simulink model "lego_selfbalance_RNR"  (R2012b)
settings: Solver=ode3  SolverMode=SingleTasking  StartTime=0.0  StopTime=100  FixedStep=0.004  MaxStep=TS  RelTol=1e-3
PostLoadFcn:
  | lego2_selfbalance_plant;
  | lego2_selfbalance_controller;
  | lego_selfbalance_simulation;
InitFcn:
  | lego2_selfbalance_plant;
  | lego2_selfbalance_controller;
  | lego_selfbalance_simulation;
  | 
  | lego_drive_selfbalance_InitData.mdl = get_param(bdroot,'Name');
  | lego_drive_selfbalance_InitData.cs = getActiveConfigSet(lego_drive_selfbalance_InitData.mdl);
model workspace: external: MAT-File (data not in the file)
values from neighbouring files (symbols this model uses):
  A1 = [    [lego2_selfbalance_plant.m]
  A2 = [    [lego2_selfbalance_plant.m]
  a_b = 0.8    [lego2_selfbalance_controller.m]
  a_d = 0.8    [lego2_selfbalance_controller.m]
  a_gc = 0.8    [lego2_selfbalance_controller.m]
  a_gd = 0.999    [lego2_selfbalance_controller.m]
  a_r = 0.996    [lego2_selfbalance_controller.m]
  B1 = [    [lego2_selfbalance_plant.m]
  B2 = [    [lego2_selfbalance_plant.m]
  BATTERY = 8000    [lego_selfbalance_simulation.m]
  C1 = eye(4)    [lego2_selfbalance_plant.m]
  C2 = eye(2)    [lego2_selfbalance_plant.m]
  D = 0.04    [lego2_selfbalance_plant.m]
  D1 = zeros(4, 2)    [lego2_selfbalance_plant.m]
  D2 = zeros(2)    [lego2_selfbalance_plant.m]
  GYRO0 = 600    [lego_selfbalance_simulation.m]
  k_f = KK(1, 1:4)    [lego2_selfbalance_controller.m]
  k_i = KK(1, 5)    [lego2_selfbalance_controller.m]
  k_sync = 0.35    [lego2_selfbalance_controller.m]
  pwm_gain = 1    [lego2_selfbalance_controller.m]
  pwm_offset = 0    [lego2_selfbalance_controller.m]
  R = 0.03    [lego2_selfbalance_plant.m]
  START_POS = [100, 100]    [lego_selfbalance_simulation.m]
  time_start = 4000    [lego2_selfbalance_controller.m]
  TS = 0.001    [lego_selfbalance_simulation.m]
  ts1 = 0.004    [lego2_selfbalance_controller.m]
  W = 0.068    [lego2_selfbalance_plant.m]
  X1IV = [    [lego_selfbalance_simulation.m]
  X2IV = [    [lego_selfbalance_simulation.m]
undefined symbols (not defined in the file or in its folder): A, DiscIntNeverNeededParam, Raw
libraries: legonxtlib x8, simulink x4

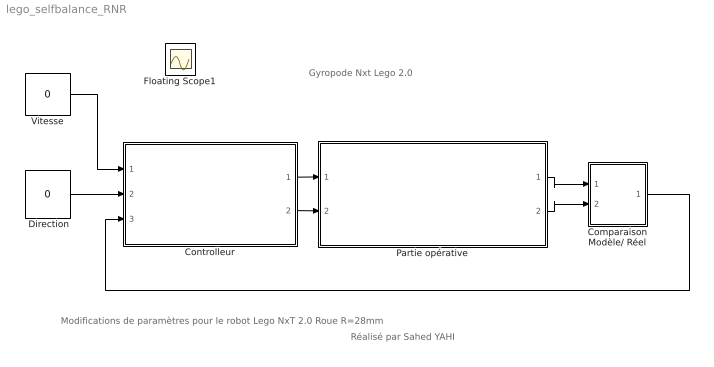
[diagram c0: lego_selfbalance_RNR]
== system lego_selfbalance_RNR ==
  note: Modifications de paramètres pour le robot Lego NxT 2.0 Roue R=28mm
  note: Réalisé par Sahed YAHI
  note: Gyropode Nxt Lego 2.0
  "   Vitesse   " : Constant  Value=0  OutDataTypeStr=single  SampleTime=4*TS
  " Direction" : Constant  Value=0  OutDataTypeStr=single  SampleTime=4*TS
  Comparaison Modèle/ Réel : Subsystem
  Controlleur : Subsystem  TreatAsAtomicUnit=on
  Partie opérative : Subsystem
  Floating Scope1 : Scope
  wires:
  "   Vitesse   "/1 -> Controlleur/1(Speed)
  " Direction"/1 -> Controlleur/2(Turn Angle)
  Controlleur/1(Right Wheel Speed) -> Partie opérative/1(R. Wheel Speed)
  Controlleur/2(Left Wheel Speed) -> Partie opérative/2(L. Wheel Speed)
  Partie opérative/1(Simulated Sensor Signals) -> Comparaison Modèle/ Réel/1(In1)
  Partie opérative/2(Actual Sensor Signals) -> Comparaison Modèle/ Réel/2(In2)
  Comparaison Modèle/ Réel/1(Out1) -> Controlleur/3(Sensor Signals)

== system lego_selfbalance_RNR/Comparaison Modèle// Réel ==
  In1 : Inport
  In2 : Inport  Port=2
  Comparaison Modèle/ Réel : simulink/Signal Routing/Environment Controller
  Out1 : Outport
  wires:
  Comparaison Modèle/ Réel/1 -> Out1/1
  In1/1 -> Comparaison Modèle/ Réel/1
  In2/1 -> Comparaison Modèle/ Réel/2

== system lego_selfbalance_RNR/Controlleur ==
  Speed : Inport
  Turn Angle : Inport  Port=2
  Sensor Signals : Inport  Port=3
  Balance and Drive Control : Subsystem
  Compare To Constant : simulink/Logic and Bit Operations/Compare To Constant  relop=>=  const=time_start  OutDataTypeStr=boolean
  Demux : Demux  Outputs=5
  Gyro Calibration : Subsystem  TreatAsAtomicUnit=on
  Logical Operator : Logic  Operator=NOT  AllPortsSameDT=off  OutDataTypeStr=boolean
  Right Wheel Speed : Outport
  Left Wheel Speed : Outport  Port=2
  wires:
  Compare To Constant/1 -> Logical Operator/1, Balance and Drive Control/Enable
  Gyro Calibration/1(Gyro Offset) -> Balance and Drive Control/1(Gyro Offset)
  Logical Operator/1 -> Gyro Calibration/Enable
  Sensor Signals/1 -> Demux/1
  Demux/4 -> Gyro Calibration/1(Gyro), Balance and Drive Control/2(Gyro)
  Speed/1 -> Balance and Drive Control/3(Speed)
  Turn Angle/1 -> Balance and Drive Control/4(Turn Angle)
  Demux/5 -> Balance and Drive Control/7(Battery)
  Demux/3 -> Balance and Drive Control/6(L. Wheel Rotation)
  Demux/2 -> Balance and Drive Control/5(R. Wheel Rotation)
  Demux/1 -> Compare To Constant/1
  Balance and Drive Control/1(R. Wheel Speed) -> Right Wheel Speed/1
  Balance and Drive Control/2(L. Wheel Speed) -> Left Wheel Speed/1

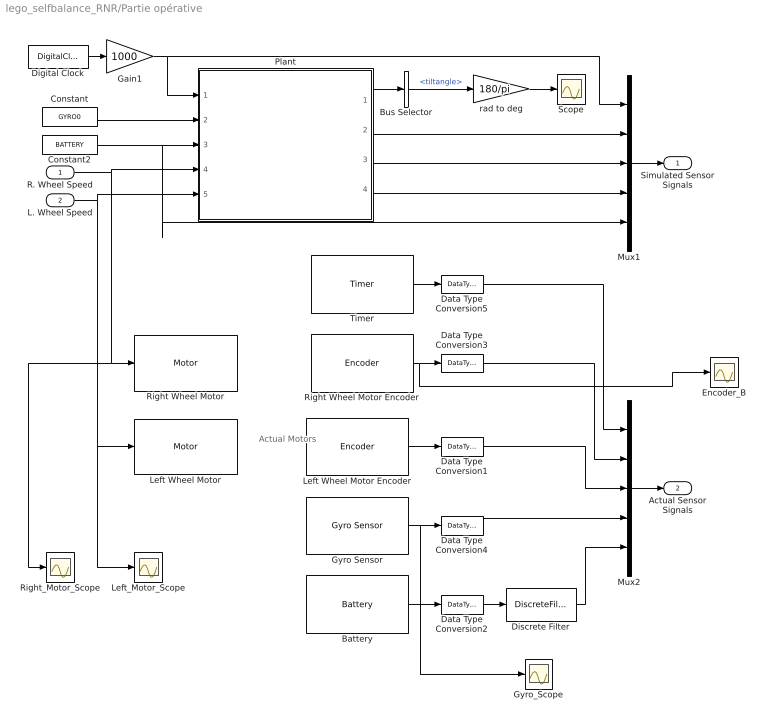
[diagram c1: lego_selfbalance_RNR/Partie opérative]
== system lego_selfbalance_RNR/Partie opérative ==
  note: Actual Motors
  R. Wheel Speed : Inport
  L. Wheel Speed : Inport  Port=2
  Battery : legonxtlib/Battery  sampleTime=ts1
  Bus Selector : BusSelector  OutputSignals=tiltangle
  Constant : Constant  Value=GYRO0  OutDataTypeStr=single
  Constant2 : Constant  Value=BATTERY  OutDataTypeStr=single
  Data Type Conversion{1..5} (5 alike) : DataTypeConversion  OutDataTypeStr=single  RndMeth=Simplest
  Digital Clock : DigitalClock  SampleTime=4*TS
  Discrete Filter : DiscreteFilter  Numerator=[1-a_b]  Denominator=[1 -a_b]
  Encoder_B : Scope
  Gain1 : Gain  Gain=1000  OutDataTypeStr=single
  Gyro Sensor : legonxtlib/Gyro Sensor  portNumber=4  outputMode=Raw A/D (0 - 1023)  offset=600  sampleTime=ts1
  Gyro_Scope : Scope
  Left Wheel Motor : legonxtlib/Motor  sportNumber=C  sstopAction=Brake
  Left Wheel Motor Encoder : legonxtlib/Encoder  portNumber=C  opMode=No reset  sampleTime=ts1
  Left_Motor_Scope : Scope
  Mux1 : Mux  Inputs=5
  Mux2 : Mux  Inputs=5
  Plant : Subsystem
  Right Wheel Motor : legonxtlib/Motor  sportNumber=B  sstopAction=Brake
  Right Wheel Motor Encoder : legonxtlib/Encoder  portNumber=B  opMode=No reset  sampleTime=ts1
  Right_Motor_Scope : Scope
  Scope : Scope
  Timer : legonxtlib/Timer  sampleTime=ts1
  rad to deg : Gain  Gain=180/pi
  Simulated Sensor Signals : Outport
  Actual Sensor Signals : Outport  Port=2
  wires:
  Data Type Conversion5/1 -> Mux2/1
  Timer/1 -> Data Type Conversion5/1
  Data Type Conversion4/1 -> Mux2/4
  Data Type Conversion1/1 -> Mux2/3
  Data Type Conversion3/1 -> Mux2/2
  Mux2/1 -> Actual Sensor Signals/1
  Left Wheel Motor Encoder/1 -> Data Type Conversion1/1
  Right Wheel Motor Encoder/1 -> Encoder_B/1, Data Type Conversion3/1
  Battery/1 -> Data Type Conversion2/1
  Data Type Conversion2/1 -> Discrete Filter/1
  Discrete Filter/1 -> Mux2/5
  Gyro Sensor/1 -> Gyro_Scope/1, Data Type Conversion4/1
  L. Wheel Speed/1 -> Plant/5(L. Wheel Speed), Left_Motor_Scope/1, Left Wheel Motor/1
  Mux1/1 -> Simulated Sensor Signals/1
  Plant/3(L. Wheel Rotation) -> Mux1/3
  Constant2/1 -> Mux1/5, Plant/3(Battery)
  Plant/2(R. Wheel Rotation) -> Mux1/2
  Plant/4(Gyro) -> Mux1/4
  Digital Clock/1 -> Gain1/1
  Gain1/1 -> Mux1/1, Plant/1(Clock)
  rad to deg/1 -> Scope/1
  Plant/1(Vertical Displacement) -> Bus Selector/1
  Bus Selector/1 -> rad to deg/1  "<tiltangle>"
  Constant/1 -> Plant/2(Gyro Offset)
  R. Wheel Speed/1 -> Plant/4(R. Wheel Speed), Right Wheel Motor/1, Right_Motor_Scope/1

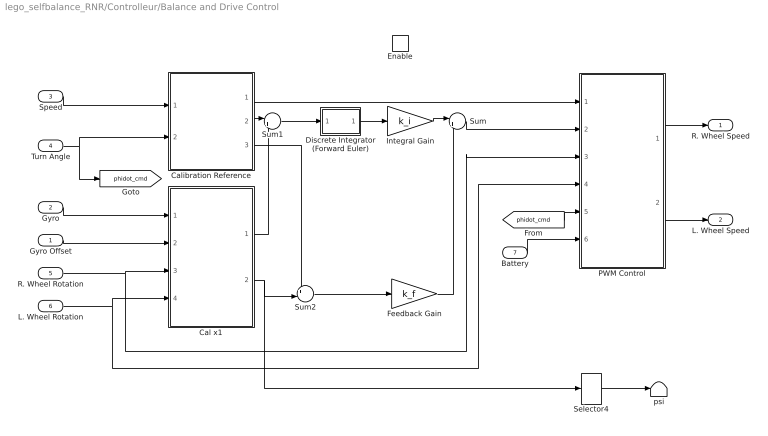
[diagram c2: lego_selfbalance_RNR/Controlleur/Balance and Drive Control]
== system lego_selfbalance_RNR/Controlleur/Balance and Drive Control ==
  Gyro Offset : Inport
  Gyro : Inport  Port=2
  Speed : Inport  Port=3
  Turn Angle : Inport  Port=4
  R. Wheel Rotation : Inport  Port=5
  L. Wheel Rotation : Inport  Port=6
  Battery : Inport  Port=7
  Enable : EnablePort
  Cal x1 : Subsystem
  Calibration Reference : Subsystem
  Discrete Integrator (Forward Euler) : Subsystem
  Feedback Gain : Gain  Gain=k_f  Multiplication=Matrix(K*u)
  Integral Gain : Gain  Gain=k_i  Multiplication=Matrix(K*u)
  PWM Control : Subsystem
  Selector4 : Selector  InputPortWidth=4  IndexOptions=Index vector (dialog)  Indices=2  OutputSizes=1
  Sum : Sum  Inputs=|++
  Sum1 : Sum  Inputs=|+-
  Sum2 : Sum  Inputs=+-|
  psi : Terminator
  R. Wheel Speed : Outport
  L. Wheel Speed : Outport  Port=2
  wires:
  [phidot_cmd] -> PWM Control/5(phidot_cmd)
  Selector4/1 -> psi/1
  Calibration Reference/3(x1_ref) -> Sum2/1
  Sum2/1 -> Feedback Gain/1
  Cal x1/2(x1) -> Selector4/1, Sum2/2
  Integral Gain/1 -> Sum/1
  Discrete Integrator (Forward Euler)/1(Out) -> Integral Gain/1
  Sum1/1 -> Discrete Integrator (Forward Euler)/1(In)
  Cal x1/1(theta) -> Sum1/2
  Calibration Reference/2(theta_ref) -> Sum1/1
  Feedback Gain/1 -> Sum/2
  L. Wheel Rotation/1 -> PWM Control/4(theta_l), Cal x1/4(L. Wheel Rotation)
  Battery/1 -> PWM Control/6(Battery)
  Sum/1 -> PWM Control/2(Voltage)
  Turn Angle/1 -> [phidot_cmd], Calibration Reference/2(Turn Angle)
  Speed/1 -> Calibration Reference/1(Speed)
  Calibration Reference/1(pwm_turn) -> PWM Control/1(pwm_turn)
  PWM Control/1(pwm_r) -> R. Wheel Speed/1
  PWM Control/2(pwm_l) -> L. Wheel Speed/1
  R. Wheel Rotation/1 -> PWM Control/3(theta_r), Cal x1/3(R. Wheel Rotation)
  Gyro/1 -> Cal x1/1(Gyro)
  Gyro Offset/1 -> Cal x1/2(Gyro Offset)

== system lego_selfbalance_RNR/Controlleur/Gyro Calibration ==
  note: Calculate gyro offset
  Gyro : Inport
  Enable : EnablePort
  Constant : Constant  Value=440  OutDataTypeStr=uint32  SampleTime=0.2
  Gain2 : Gain  Gain=1-a_gc
  Gain3 : Gain  Gain=a_gc
  Speaker : legonxtlib/Speaker  sinputMode=Frequency only  sspeakerFreq=100  sspeakerVolume=80  sspeakerDuration=100
  Sum1 : Sum  Inputs=|++
  Unit Delay : UnitDelay  SampleTime=-1
  Gyro Offset : Outport
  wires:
  Gain3/1 -> Sum1/2
  Unit Delay/1 -> Gain3/1
  Sum1/1 -> Unit Delay/1, Gyro Offset/1
  Gain2/1 -> Sum1/1
  Gyro/1 -> Gain2/1
  Constant/1 -> Speaker/1

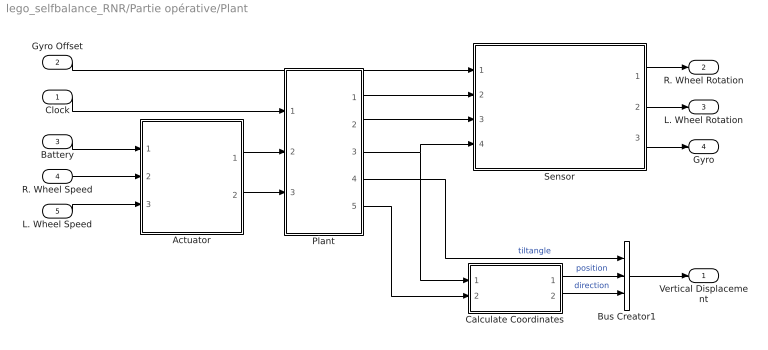
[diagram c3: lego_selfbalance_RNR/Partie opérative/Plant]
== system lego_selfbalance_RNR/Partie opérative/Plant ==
  Clock : Inport
  Gyro Offset : Inport  Port=2
  Battery : Inport  Port=3
  R. Wheel Speed : Inport  Port=4
  L. Wheel Speed : Inport  Port=5
  Actuator : Subsystem
  Bus Creator1 : BusCreator  Inputs=3
  Calculate Coordinates : Subsystem
  Plant : Subsystem
  Sensor : Subsystem
  Vertical Displacement : Outport
  R. Wheel Rotation : Outport  Port=2
  L. Wheel Rotation : Outport  Port=3
  Gyro : Outport  Port=4
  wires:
  Clock/1 -> Plant/1(Clock)
  Plant/4(psi) -> Bus Creator1/1  "tiltangle"
  Bus Creator1/1 -> Vertical Displacement/1
  Calculate Coordinates/2(direction) -> Bus Creator1/3  "direction"
  Calculate Coordinates/1(position) -> Bus Creator1/2  "position"
  Plant/3(phi) -> Calculate Coordinates/1(phi), Sensor/4(phi)
  L. Wheel Speed/1 -> Actuator/3(L. Wheel Speed)
  Plant/5(thetadot) -> Calculate Coordinates/2(thetadot)
  Sensor/3(Gyro) -> Gyro/1
  R. Wheel Speed/1 -> Actuator/2(R. Wheel Speed)
  Sensor/2(L. Wheel Rotation) -> L. Wheel Rotation/1
  Sensor/1(R. Wheel Rotation) -> R. Wheel Rotation/1
  Gyro Offset/1 -> Sensor/1(Gyro Offset)
  Battery/1 -> Actuator/1(Battery)
  Plant/1(theta) -> Sensor/2(theta)
  Plant/2(psidot) -> Sensor/3(psidot)
  Actuator/2(vol_l) -> Plant/3(vol_l)
  Actuator/1(vol_r) -> Plant/2(vol_r)

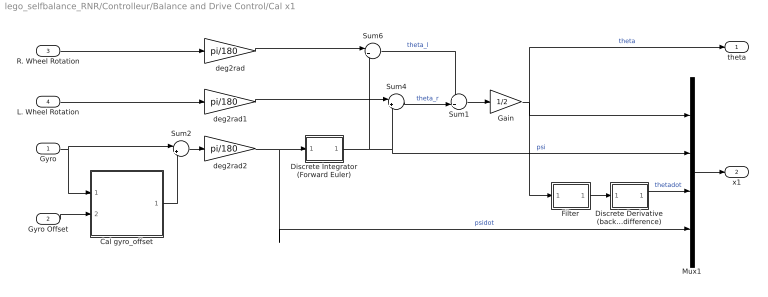
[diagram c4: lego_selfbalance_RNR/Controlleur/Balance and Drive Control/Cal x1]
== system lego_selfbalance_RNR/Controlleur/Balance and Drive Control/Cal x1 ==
  Gyro : Inport
  Gyro Offset : Inport  Port=2
  R. Wheel Rotation : Inport  Port=3
  L. Wheel Rotation : Inport  Port=4
  Cal gyro_offset : Subsystem
  Discrete Derivative (backward difference) : Subsystem
  Discrete Integrator (Forward Euler) : Subsystem
  Filter : Subsystem
  Gain : Gain  Gain=1/2
  Mux1 : Mux
  Sum1 : Sum  Inputs=++|
  Sum2 : Sum  Inputs=|+-
  Sum4 : Sum  Inputs=|++
  Sum6 : Sum  Inputs=|++
  deg2rad : Gain  Gain=pi/180
  deg2rad1 : Gain  Gain=pi/180
  deg2rad2 : Gain  Gain=pi/180
  theta : Outport
  x1 : Outport  Port=2
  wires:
  Gain/1 -> Mux1/1, theta/1, Filter/1(In)  "theta"
  Filter/1(Out) -> Discrete Derivative (backward difference)/1(In)
  deg2rad2/1 -> Mux1/4, Discrete Integrator (Forward Euler)/1(in)  "psidot"
  Sum1/1 -> Gain/1
  Sum4/1 -> Sum1/2  "theta_r"
  Sum6/1 -> Sum1/1  "theta_l"
  Discrete Derivative (backward difference)/1(Out) -> Mux1/3  "thetadot"
  L. Wheel Rotation/1 -> deg2rad1/1
  R. Wheel Rotation/1 -> deg2rad/1
  deg2rad/1 -> Sum6/1
  Discrete Integrator (Forward Euler)/1(out) -> Mux1/2, Sum4/2, Sum6/2  "psi"
  Mux1/1 -> x1/1
  deg2rad1/1 -> Sum4/1
  Gyro/1 -> Sum2/1, Cal gyro_offset/1(Gyro)
  Sum2/1 -> deg2rad2/1
  Cal gyro_offset/1(Gyro Offset) -> Sum2/2
  Gyro Offset/1 -> Cal gyro_offset/2(Gyro Offset 0)

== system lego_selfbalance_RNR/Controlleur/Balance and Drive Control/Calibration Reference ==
  note: thetadot_cmd should be between 0 and 7.5
  note: phidot_cmd should be between 0 and 25
  Speed : Inport
  Turn Angle : Inport  Port=2
  Constant2 : Constant  Value=0  VectorParams1D=off  OutDataTypeStr=single
  Constant3 : Constant  Value=0  VectorParams1D=off  OutDataTypeStr=single
  Discrete Integrator (Forward Euler) : Subsystem
  Filter : Subsystem
  Mux : Mux
  pwm_turn : Outport
  theta_ref : Outport  Port=2
  x1_ref : Outport  Port=3
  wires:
  Filter/1(out) -> Mux/3, Discrete Integrator (Forward Euler)/1(in)  "thetadot_ref"
  Constant3/1 -> Mux/4  "psidot_ref"
  Constant2/1 -> Mux/2  "psi_ref"
  Discrete Integrator (Forward Euler)/1(out) -> Mux/1, theta_ref/1  "theta_ref"
  Mux/1 -> x1_ref/1
  Turn Angle/1 -> pwm_turn/1
  Speed/1 -> Filter/1(in)

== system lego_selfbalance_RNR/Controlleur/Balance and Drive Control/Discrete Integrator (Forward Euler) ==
  In : Inport
  Gain : Gain  Gain=ts1
  Sum : Sum  Inputs=|++
  Unit Delay : UnitDelay  SampleTime=-1
  Out : Outport
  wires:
  In/1 -> Gain/1
  Sum/1 -> Unit Delay/1
  Gain/1 -> Sum/1
  Unit Delay/1 -> Out/1, Sum/2

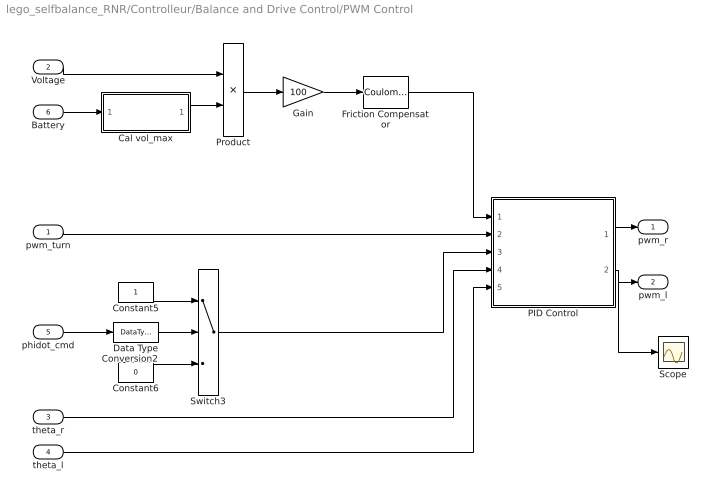
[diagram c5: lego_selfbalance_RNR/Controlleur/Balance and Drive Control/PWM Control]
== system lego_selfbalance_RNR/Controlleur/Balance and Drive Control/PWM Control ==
  pwm_turn : Inport
  Voltage : Inport  Port=2
  theta_r : Inport  Port=3
  theta_l : Inport  Port=4
  phidot_cmd : Inport  Port=5
  Battery : Inport  Port=6
  Cal vol_max : Subsystem
  Constant5 : Constant  OutDataTypeStr=boolean
  Constant6 : Constant  Value=0  OutDataTypeStr=boolean
  Data Type Conversion2 : DataTypeConversion  OutDataTypeStr=int8  RndMeth=Simplest
  Friction Compensator : simulink/Discontinuities/Coulomb & Viscous Friction  offset=pwm_offset  gain=pwm_gain
  Gain : Gain  Gain=100
  PID Control : Subsystem
  Product : Product  Inputs=*/  RndMeth=Simplest
  Scope : Scope
  Switch3 : Switch  Criteria=u2 ~= 0
  pwm_r : Outport
  pwm_l : Outport  Port=2
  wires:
  Data Type Conversion2/1 -> Switch3/2
  phidot_cmd/1 -> Data Type Conversion2/1
  Constant6/1 -> Switch3/3
  Constant5/1 -> Switch3/1
  theta_l/1 -> PID Control/5(In5)
  theta_r/1 -> PID Control/4(In4)
  Cal vol_max/1(vol_max) -> Product/2
  Battery/1 -> Cal vol_max/1(battery)
  Product/1 -> Gain/1
  Voltage/1 -> Product/1
  Gain/1 -> Friction Compensator/1
  PID Control/1(pwm_r) -> pwm_r/1
  Friction Compensator/1 -> PID Control/1(In1)
  PID Control/2(pwm_l) -> Scope/1, pwm_l/1
  pwm_turn/1 -> PID Control/2(In2)
  Switch3/1 -> PID Control/3(In3)

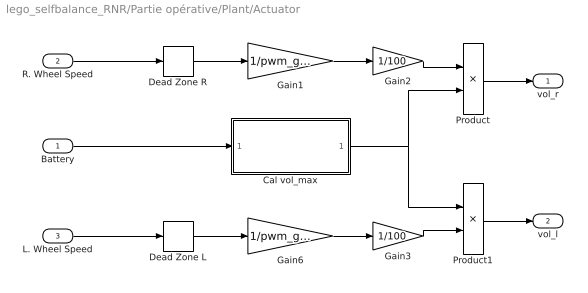
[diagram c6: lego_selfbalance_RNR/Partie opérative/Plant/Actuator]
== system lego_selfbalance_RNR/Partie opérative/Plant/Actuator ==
  Battery : Inport
  R. Wheel Speed : Inport  Port=2
  L. Wheel Speed : Inport  Port=3
  Cal vol_max : Subsystem
  Dead Zone L : DeadZone  LowerValue=-pwm_offset  UpperValue=pwm_offset
  Dead Zone R : DeadZone  LowerValue=-pwm_offset  UpperValue=pwm_offset
  Gain1 : Gain  Gain=1/pwm_gain
  Gain2 : Gain  Gain=1/100
  Gain3 : Gain  Gain=1/100
  Gain6 : Gain  Gain=1/pwm_gain
  Product : Product  RndMeth=Simplest
  Product1 : Product  RndMeth=Simplest
  vol_r : Outport
  vol_l : Outport  Port=2
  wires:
  Battery/1 -> Cal vol_max/1(Battery)
  Cal vol_max/1(vol_max) -> Product1/1, Product/2
  Dead Zone R/1 -> Gain1/1
  Product1/1 -> vol_l/1
  Gain3/1 -> Product1/2
  Product/1 -> vol_r/1
  Gain2/1 -> Product/1
  Gain6/1 -> Gain3/1
  Gain1/1 -> Gain2/1
  L. Wheel Speed/1 -> Dead Zone L/1
  R. Wheel Speed/1 -> Dead Zone R/1
  Dead Zone L/1 -> Gain6/1

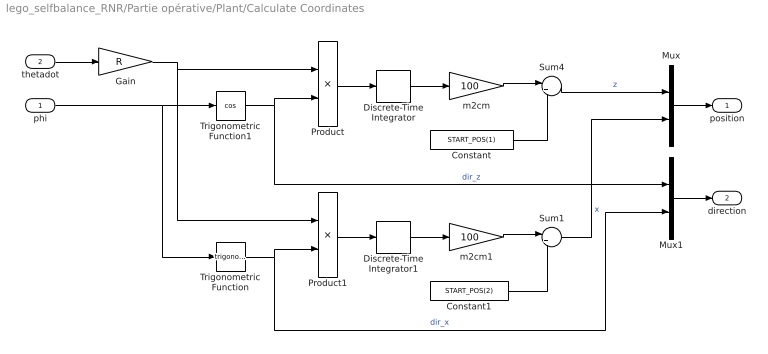
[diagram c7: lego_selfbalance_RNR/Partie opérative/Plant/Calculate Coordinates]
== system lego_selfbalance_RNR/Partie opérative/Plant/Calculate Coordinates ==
  phi : Inport
  thetadot : Inport  Port=2
  Constant : Constant  Value=START_POS(1)  OutDataTypeStr=double
  Constant1 : Constant  Value=START_POS(2)  OutDataTypeStr=double
  Discrete-Time Integrator : DiscreteIntegrator  SampleTime=4*TS  ICPrevOutput=DiscIntNeverNeededParam  ICPrevScaledInput=DiscIntNeverNeededParam
  Discrete-Time Integrator1 : DiscreteIntegrator  SampleTime=4*TS  ICPrevOutput=DiscIntNeverNeededParam  ICPrevScaledInput=DiscIntNeverNeededParam
  Gain : Gain  Gain=R
  Mux : Mux  Inputs=2
  Mux1 : Mux  Inputs=2
  Product : Product  OutDataTypeStr=double  RndMeth=Simplest
  Product1 : Product  OutDataTypeStr=double  RndMeth=Simplest
  Sum1 : Sum  Inputs=|++
  Sum4 : Sum  Inputs=|++
  Trigonometric Function : Trigonometry
  Trigonometric Function1 : Trigonometry  Operator=cos
  m2cm : Gain  Gain=100
  m2cm1 : Gain  Gain=100
  position : Outport
  direction : Outport  Port=2
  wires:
  Mux1/1 -> direction/1
  Mux/1 -> position/1
  Sum1/1 -> Mux/2  "x"
  Constant1/1 -> Sum1/2
  m2cm1/1 -> Sum1/1
  Constant/1 -> Sum4/2
  Sum4/1 -> Mux/1  "z"
  m2cm/1 -> Sum4/1
  Gain/1 -> Product/1, Product1/1
  Discrete-Time Integrator1/1 -> m2cm1/1
  Discrete-Time Integrator/1 -> m2cm/1
  phi/1 -> Trigonometric Function/1, Trigonometric Function1/1
  thetadot/1 -> Gain/1
  Trigonometric Function1/1 -> Mux1/1, Product/2  "dir_z"
  Product/1 -> Discrete-Time Integrator/1
  Trigonometric Function/1 -> Mux1/2, Product1/2  "dir_x"
  Product1/1 -> Discrete-Time Integrator1/1

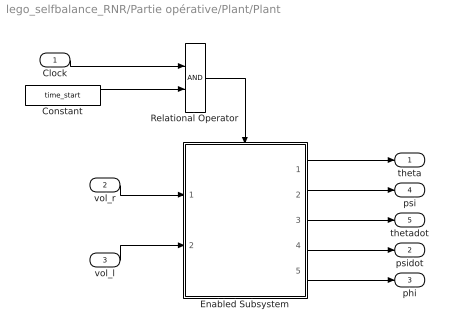
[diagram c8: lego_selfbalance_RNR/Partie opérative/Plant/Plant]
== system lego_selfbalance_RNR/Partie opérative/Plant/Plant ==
  Clock : Inport
  vol_r : Inport  Port=2
  vol_l : Inport  Port=3
  Constant : Constant  Value=time_start  OutDataTypeStr=single
  Enabled Subsystem : Subsystem  TreatAsAtomicUnit=on
  Relational Operator : RelationalOperator  OutDataTypeStr=boolean
  theta : Outport
  psidot : Outport  Port=2
  phi : Outport  Port=3
  psi : Outport  Port=4
  thetadot : Outport  Port=5
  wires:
  Enabled Subsystem/4(psidot) -> psidot/1
  Enabled Subsystem/5(phi) -> phi/1
  Enabled Subsystem/2(psi) -> psi/1
  Enabled Subsystem/3(thetadot) -> thetadot/1
  Enabled Subsystem/1(theta) -> theta/1
  Constant/1 -> Relational Operator/2
  Clock/1 -> Relational Operator/1
  Relational Operator/1 -> Enabled Subsystem/Enable
  vol_l/1 -> Enabled Subsystem/2(vol_l)
  vol_r/1 -> Enabled Subsystem/1(vol_r)

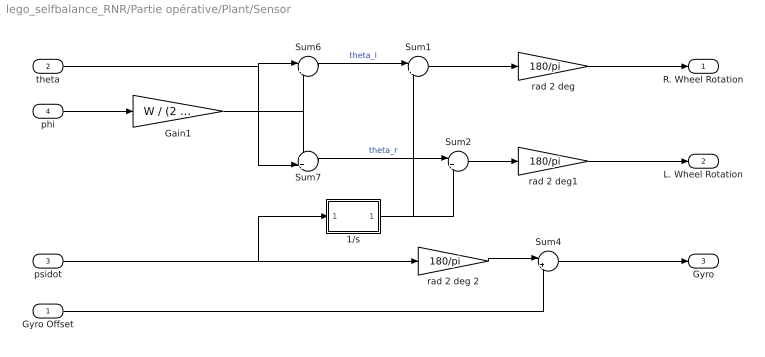
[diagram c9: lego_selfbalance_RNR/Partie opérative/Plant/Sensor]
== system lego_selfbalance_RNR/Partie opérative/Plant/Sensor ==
  Gyro Offset : Inport
  theta : Inport  Port=2
  psidot : Inport  Port=3
  phi : Inport  Port=4
  1/s : Subsystem
  Gain1 : Gain  Gain=W / (2 * R)
  Sum1 : Sum  Inputs=|+-
  Sum2 : Sum  Inputs=|+-
  Sum4 : Sum  Inputs=|++
  Sum6 : Sum  Inputs=|+-
  Sum7 : Sum  Inputs=++|
  rad 2 deg : Gain  Gain=180/pi  OutDataTypeStr=single
  rad 2 deg 2 : Gain  Gain=180/pi
  rad 2 deg1 : Gain  Gain=180/pi  OutDataTypeStr=single
  R. Wheel Rotation : Outport
  L. Wheel Rotation : Outport  Port=2
  Gyro : Outport  Port=3
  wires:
  1/s/1(Out1) -> Sum1/2, Sum2/2
  Sum6/1 -> Sum1/1  "theta_l"
  rad 2 deg1/1 -> L. Wheel Rotation/1
  rad 2 deg/1 -> R. Wheel Rotation/1
  Sum2/1 -> rad 2 deg1/1
  psidot/1 -> 1/s/1(In1), rad 2 deg 2/1
  Sum1/1 -> rad 2 deg/1
  Gain1/1 -> Sum6/2, Sum7/1
  phi/1 -> Gain1/1
  theta/1 -> Sum6/1, Sum7/2
  rad 2 deg 2/1 -> Sum4/1
  Sum7/1 -> Sum2/1  "theta_r"
  Gyro Offset/1 -> Sum4/2
  Sum4/1 -> Gyro/1

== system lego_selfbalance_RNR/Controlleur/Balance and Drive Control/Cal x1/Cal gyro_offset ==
  Gyro : Inport
  Gyro Offset 0 : Inport  Port=2
  Gain1 : Gain  Gain=1-a_gd
  Gain4 : Gain  Gain=a_gd
  Sum2 : Sum  Inputs=|++
  Unit Delay External IC : simulink/Additional Math & Discrete/Additional Discrete/Unit Delay External IC  tsamp=-1
  Gyro Offset : Outport
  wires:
  Gyro/1 -> Gain1/1
  Gyro Offset 0/1 -> Unit Delay External IC/2
  Gain1/1 -> Sum2/1
  Sum2/1 -> Gyro Offset/1, Unit Delay External IC/1
  Unit Delay External IC/1 -> Gain4/1
  Gain4/1 -> Sum2/2

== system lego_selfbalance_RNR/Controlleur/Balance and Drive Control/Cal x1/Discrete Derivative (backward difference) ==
  In : Inport
  Gain : Gain  Gain=1/ts1
  Sum : Sum  Inputs=|+-
  Unit Delay : UnitDelay  SampleTime=-1
  Out : Outport
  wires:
  Gain/1 -> Out/1
  In/1 -> Sum/1, Unit Delay/1
  Unit Delay/1 -> Sum/2
  Sum/1 -> Gain/1

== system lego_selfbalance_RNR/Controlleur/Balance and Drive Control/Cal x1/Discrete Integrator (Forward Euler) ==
  in : Inport
  Gain : Gain  Gain=ts1
  Sum : Sum  Inputs=|++
  Unit Delay : UnitDelay  SampleTime=-1
  out : Outport
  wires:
  Unit Delay/1 -> Sum/2, out/1
  Gain/1 -> Sum/1
  Sum/1 -> Unit Delay/1
  in/1 -> Gain/1

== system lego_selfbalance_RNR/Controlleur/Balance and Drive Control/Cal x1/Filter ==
  In : Inport
  Gain2 : Gain  Gain=a_d
  Gain3 : Gain  Gain=1-a_d
  Sum : Sum  Inputs=|++
  Unit Delay : UnitDelay  SampleTime=-1
  Out : Outport
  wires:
  In/1 -> Gain3/1
  Gain3/1 -> Sum/1
  Gain2/1 -> Sum/2
  Unit Delay/1 -> Gain2/1
  Sum/1 -> Out/1, Unit Delay/1

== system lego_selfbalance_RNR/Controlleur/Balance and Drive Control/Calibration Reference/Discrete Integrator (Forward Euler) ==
  in : Inport
  Gain : Gain  Gain=ts1
  Sum : Sum  Inputs=|++
  Unit Delay : UnitDelay  SampleTime=-1
  out : Outport
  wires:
  in/1 -> Gain/1
  Sum/1 -> Unit Delay/1
  Gain/1 -> Sum/1
  Unit Delay/1 -> out/1, Sum/2

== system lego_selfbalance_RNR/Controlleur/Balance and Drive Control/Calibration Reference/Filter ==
  note: Filter Function: 1-a_r ---------------- 1-a_r*z^(-1)
  in : Inport
  Gain2 : Gain  Gain=a_r
  Gain3 : Gain  Gain=1-a_r
  Sum : Sum  Inputs=|++
  Unit Delay : UnitDelay  SampleTime=-1
  out : Outport
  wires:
  in/1 -> Gain3/1
  Gain3/1 -> Sum/1
  Gain2/1 -> Sum/2
  Unit Delay/1 -> Gain2/1
  Sum/1 -> out/1, Unit Delay/1

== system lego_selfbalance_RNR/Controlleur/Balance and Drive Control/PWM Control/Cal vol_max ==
  battery : Inport
  Constant : Constant  Value=0.625  OutDataTypeStr=single
  Gain3 : Gain  Gain=0.001089
  Sum2 : Sum  Inputs=|+-
  vol_max : Outport
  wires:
  Gain3/1 -> Sum2/1
  Sum2/1 -> vol_max/1
  Constant/1 -> Sum2/2
  battery/1 -> Gain3/1

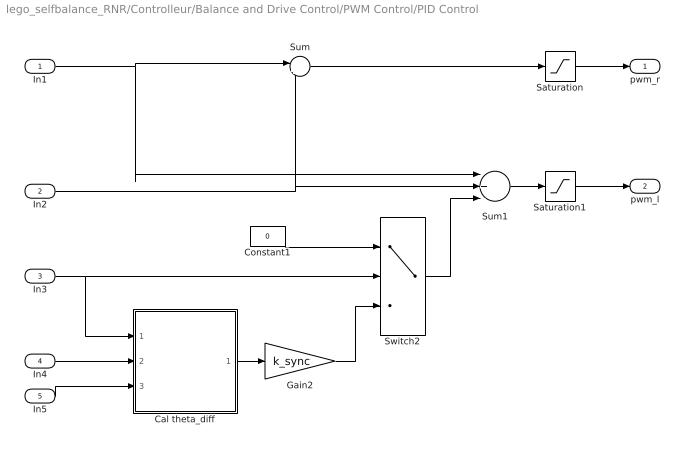
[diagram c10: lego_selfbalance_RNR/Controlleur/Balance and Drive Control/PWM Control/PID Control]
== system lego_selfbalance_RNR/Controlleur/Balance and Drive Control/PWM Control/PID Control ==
  In1 : Inport
  In2 : Inport  Port=2
  In3 : Inport  Port=3
  In4 : Inport  Port=4
  In5 : Inport  Port=5
  Cal theta_diff : Subsystem
  Constant1 : Constant  Value=0  OutDataTypeStr=single
  Gain2 : Gain  Gain=k_sync
  Saturation : Saturate  UpperLimit=100  LowerLimit=-100
  Saturation1 : Saturate  UpperLimit=100  LowerLimit=-100
  Sum : Sum  Inputs=|++
  Sum1 : Sum  Inputs=|+-+
  Switch2 : Switch  Criteria=u2 ~= 0
  pwm_r : Outport
  pwm_l : Outport  Port=2
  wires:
  In1/1 -> Sum1/1, Sum/1
  Gain2/1 -> Switch2/3
  Constant1/1 -> Switch2/1
  In3/1 -> Switch2/2, Cal theta_diff/1(flag_turn)
  Cal theta_diff/1(theta_diff) -> Gain2/1
  Saturation/1 -> pwm_r/1
  Saturation1/1 -> pwm_l/1
  In2/1 -> Sum1/2, Sum/2
  Sum/1 -> Saturation/1
  In4/1 -> Cal theta_diff/2(theta_r)
  In5/1 -> Cal theta_diff/3(theta_l)
  Switch2/1 -> Sum1/3
  Sum1/1 -> Saturation1/1

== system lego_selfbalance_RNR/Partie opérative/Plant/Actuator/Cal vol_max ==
  note: Calculate maximum DC motor (battery) voltage using an experimental expression
  Battery : Inport
  Constant : Constant  Value=0.625  OutDataTypeStr=single
  Gain3 : Gain  Gain=0.001089
  Sum2 : Sum  Inputs=|+-
  vol_max : Outport
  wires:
  Constant/1 -> Sum2/2
  Sum2/1 -> vol_max/1
  Gain3/1 -> Sum2/1
  Battery/1 -> Gain3/1

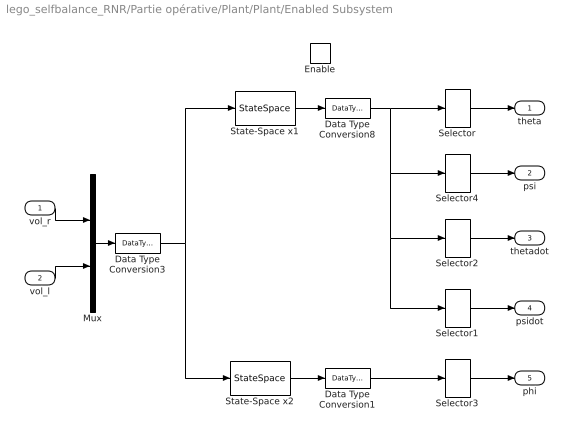
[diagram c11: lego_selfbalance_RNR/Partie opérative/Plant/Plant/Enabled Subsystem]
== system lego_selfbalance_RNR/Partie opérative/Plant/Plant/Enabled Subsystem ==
  vol_r : Inport
  vol_l : Inport  Port=2
  Enable : EnablePort
  Data Type Conversion1 : DataTypeConversion  OutDataTypeStr=single  RndMeth=Nearest
  Data Type Conversion3 : DataTypeConversion  OutDataTypeStr=double  RndMeth=Nearest
  Data Type Conversion8 : DataTypeConversion  OutDataTypeStr=single  RndMeth=Nearest
  Mux : Mux  Inputs=2
  Selector : Selector  InputPortWidth=4  IndexOptions=Index vector (dialog)  Indices=1  OutputSizes=1
  Selector1 : Selector  InputPortWidth=4  IndexOptions=Index vector (dialog)  Indices=4  OutputSizes=1
  Selector2 : Selector  InputPortWidth=4  IndexOptions=Index vector (dialog)  Indices=3  OutputSizes=1
  Selector3 : Selector  InputPortWidth=2  IndexOptions=Index vector (dialog)  Indices=1  OutputSizes=1
  Selector4 : Selector  InputPortWidth=4  IndexOptions=Index vector (dialog)  Indices=2  OutputSizes=1
  State-Space x1 : StateSpace  A=A1  B=B1  C=C1  D=D1  X0=X1IV
  State-Space x2 : StateSpace  A=A2  B=B2  C=C2  D=D2  X0=X2IV
  theta : Outport  InitialOutput=0
  psi : Outport  Port=2  InitialOutput=0
  thetadot : Outport  Port=3  InitialOutput=0
  psidot : Outport  Port=4  InitialOutput=0
  phi : Outport  Port=5  InitialOutput=0
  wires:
  Data Type Conversion1/1 -> Selector3/1
  Data Type Conversion3/1 -> State-Space x1/1, State-Space x2/1
  Data Type Conversion8/1 -> Selector2/1, Selector1/1, Selector4/1, Selector/1
  Selector1/1 -> psidot/1
  Selector/1 -> theta/1
  Selector4/1 -> psi/1
  Selector2/1 -> thetadot/1
  Selector3/1 -> phi/1
  Mux/1 -> Data Type Conversion3/1
  vol_l/1 -> Mux/2
  vol_r/1 -> Mux/1
  State-Space x1/1 -> Data Type Conversion8/1
  State-Space x2/1 -> Data Type Conversion1/1

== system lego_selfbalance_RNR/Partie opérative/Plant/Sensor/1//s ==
  In1 : Inport
  Data Type Conversion1 : DataTypeConversion  OutDataTypeStr=double  RndMeth=Nearest
  Discrete-Time Integrator : DiscreteIntegrator  gainval=1  SampleTime=4*TS  ICPrevOutput=DiscIntNeverNeededParam  ICPrevScaledInput=DiscIntNeverNeededParam
  Out1 : Outport
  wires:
  In1/1 -> Data Type Conversion1/1
  Data Type Conversion1/1 -> Discrete-Time Integrator/1
  Discrete-Time Integrator/1 -> Out1/1

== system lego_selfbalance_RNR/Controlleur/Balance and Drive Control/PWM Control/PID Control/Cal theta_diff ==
  note: Save the difference between left and right motor revolution angle
  note: Detect turn -> straight run change
  note: When phidot goes to 0, remember the difference between L and R encoder values (they need not be equal, since robot would have been turning). While phidot == 0, apply correction to maintain that difference. If phidot ~= 0, don't apply the correction.
  flag_turn : Inport
  theta_r : Inport  Port=2
  theta_l : Inport  Port=3
  Detect Flag Falling : Subsystem
  Set theta_offset : Subsystem
  Sum1 : Sum  Inputs=|+-
  Sum5 : Sum  Inputs=|-+
  theta_diff : Outport
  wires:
  Set theta_offset/1(theta_offset) -> Sum5/1
  theta_l/1 -> Sum1/2
  theta_r/1 -> Sum1/1
  Sum1/1 -> Sum5/2, Set theta_offset/1(theta_diff)
  Detect Flag Falling/1(falling) -> Set theta_offset/Enable
  Sum5/1 -> theta_diff/1
  flag_turn/1 -> Detect Flag Falling/1(flag)

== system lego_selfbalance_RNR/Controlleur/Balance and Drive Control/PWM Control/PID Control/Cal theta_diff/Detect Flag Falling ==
  flag : Inport
  Constant : Constant  Value=0  VectorParams1D=off  OutDataTypeStr=boolean
  Constant1 : Constant  VectorParams1D=off  OutDataTypeStr=boolean
  Logical Operator : Logic  AllPortsSameDT=off  OutDataTypeStr=boolean
  Relational Operator : RelationalOperator  Operator===  OutDataTypeStr=boolean
  Relational Operator1 : RelationalOperator  Operator===  OutDataTypeStr=boolean
  Unit Delay : UnitDelay  SampleTime=-1
  falling : Outport
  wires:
  Logical Operator/1 -> falling/1
  Relational Operator1/1 -> Logical Operator/2
  Relational Operator/1 -> Logical Operator/1
  Constant1/1 -> Relational Operator1/2
  Unit Delay/1 -> Relational Operator1/1
  Constant/1 -> Relational Operator/2
  flag/1 -> Relational Operator/1, Unit Delay/1

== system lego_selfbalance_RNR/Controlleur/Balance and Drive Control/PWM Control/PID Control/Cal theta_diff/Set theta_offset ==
  theta_diff : Inport
  Enable : EnablePort
  theta_offset : Outport
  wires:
  theta_diff/1 -> theta_offset/1
